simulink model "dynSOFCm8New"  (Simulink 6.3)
settings: Solver=ode15s  StartTime=0.0  StopTime=5000  FixedStep=0.001  MinStep=1e-12  RelTol=1e-3
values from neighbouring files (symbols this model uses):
  C = 300e-2    (= 3)    [dynSOFC_par.m]
  Cpc = 740    [dynSOFC_par.m]
  Cpt = 1217.7    [dynSOFC_par.m]
  D_a = 0.273*2*r3    (= 0.006006)    [dynSOFC_par.m]
  D_c = 2*(r2-r1)    (= 0.00532)    [dynSOFC_par.m]
  delta = 5.67e-8    (= 5.67e-08)    [dynSOFC_par.m]
  Ea = 1.1e5    (= 110000)    [dynSOFC_par.m]
  Ec = 1.2e5    (= 120000)    [dynSOFC_par.m]
  Ems1 = 0.4    [dynSOFC_par.m]
  Ems2 = 0.9    [dynSOFC_par.m]
  F = 96487    [dynSOFC_par.m]
  F21 = 0.69    [dynSOFC_par.m]
  K = 10    [dynSOFC_par.m]
  L = 1.5    [dynSOFC_par.m]
  La = 0.1e-3    (= 0.0001)    [dynSOFC_par.m]
  Lc = 2.21e-3    (= 0.00221)    [dynSOFC_par.m]
  Le = 0.04e-3    (= 4e-05)    [dynSOFC_par.m]
  R = 8.314/101325    (= 8.20528003948e-05)    [dynSOFC_par.m]
  r0 = 5e-3    (= 0.005)    [dynSOFC_par.m]
  r1 = 6e-3    (= 0.006)    [dynSOFC_par.m]
  r2 = 8.66e-3    (= 0.00866)    [dynSOFC_par.m]
  r3 = 11e-3    (= 0.011)    [dynSOFC_par.m]
  Ro = 1e-6    (= 1e-06)    [dynSOFC_par.m]
  Rouc = 4592    [dynSOFC_par.m]
  Rout = 3900    [dynSOFC_par.m]
  X = z(i)    [Simulate.m]    (also in dynSOFC_par.m = 0)
  x_ini = x_INI(i,:)    [Simulate.m]    (also in dynSOFC_par.m = [)
  XCH4 = 0.173    [dynSOFC_par.m]
  XCO = 0.057    [dynSOFC_par.m]
  XCO2 = 0.228    [dynSOFC_par.m]
  XH2 = 0.258    [dynSOFC_par.m]
  XH2O = 0.284    [dynSOFC_par.m]
  XO2 = 0.21    [dynSOFC_par.m]
libraries: simulink x23
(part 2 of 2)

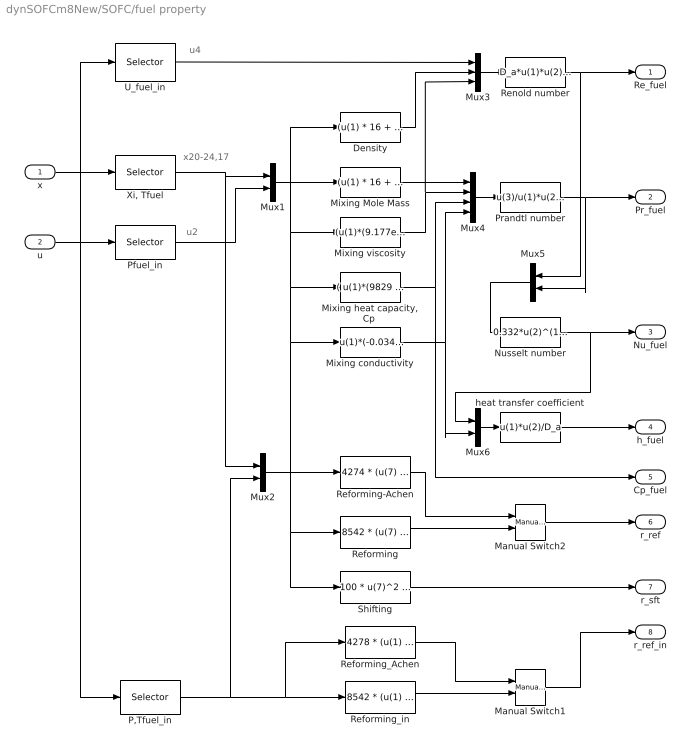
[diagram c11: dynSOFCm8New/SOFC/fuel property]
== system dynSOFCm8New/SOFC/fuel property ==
  note: x20-24,17
  note: u4
  note: u2
  x : Inport
  u : Inport  Port=2
  Density : Fcn  Expr="(u(1) * 16 + u(2) * 18 + u(3) * 2 + u(4) *28 + u(5) *44)  * u(7)/(R*u(6)) / 1000"
  Manual Switch1 : simulink/Signal Routing/Manual Switch  sw=0  action=0
  Manual Switch2 : simulink/Signal Routing/Manual Switch  sw=0  action=0
  Mixing Mole Mass : Fcn  Expr=(u(1) * 16 + u(2) * 18 + u(3) * 2 + u(4) *28 + u(5) *44)
  Mixing conductivity : Fcn  Expr=u(1)*(-0.03442 + 1.987e-4*u(6)) + u(2)*(-0.01450 + 9.782e-5*u(6)) + u(3)*(0.08525 + 2.964e-4*u(6)) + u(4)*(0.01275 + 5.348e-5*u(6)) + u(5)*(0.005485 + 6.272e-5*u(6))
  "Mixing heat capacity, Cp " : Fcn  Expr="( u(1)*(9829 + 83.47*u(6) -0.02053*u(6)^2)  + u(2)*(2.906e4 + 12.15*u(6)) +  u(3)*(2.660e4 +3.719*u(6)) + u(4)*(2.797e4 + 5.019*u(6)) + u(5)*(3.200e4 + 31.01*u(6) - 0.008875*u(6)^2) )"
  Mixing viscosity : Fcn  Expr="(u(1)*(9.177e-6 + 1.755e-8*u(6)) +  u(2)*(4.567e-6 + 2.209e-8*u(6)) + u(3)*(6.162e-6 + 1.145e-8*u(6)) + u(4)*(1.399e-5 + 2.582e-8*u(6)) + u(5)*(1.273e-5 + 2.822e-8*u(6)) )"
  Mux1 : Mux  Inputs=2
  Mux2 : Mux  Inputs=2
  Mux3 : Mux  Inputs=3
  Mux4 : Mux
  Mux5 : Mux  Orientation=left  Inputs=2
  Mux6 : Mux  Inputs=2
  Nusselt number : Fcn  Expr=0.332*u(2)^(1/3)*u(1)^(1/2)
  P,Tfuel_in : Selector  Elements=[2 3]  InputPortWidth=7
  Pfuel_in : Selector  Elements=[2]  InputPortWidth=7
  Prandtl number : Fcn  Expr=u(3)/u(1)*u(2)/u(4)
  Reforming : Fcn  Expr=8542 * (u(7) * u(1))^(0.85) * (u(7) * u(2))^(-0.35) * exp( -95e3 /(8.314*u(6)) )
  Reforming-Achen : Fcn  Expr=4274 * (u(7) * u(1)) * exp( -82e3 /(8.314*u(6)) )
  Reforming_Achen : Fcn  Expr=4278 * (u(1) * XCH4) * exp( -82e3 /(8.314*u(2)) )
  Reforming_in : Fcn  Expr=8542 * (u(1) * XCH4)^(0.85) * (u(1) * XH2O)^(-0.35) * exp( -95e3 /(8.314*u(2)) )
  Renold number : Fcn  Expr=D_a*u(1)*u(2)/u(3)
  Shifting : Fcn  Expr="100 * u(7)^2 * ( exp( 4276/u(6) - 3.961 ) * u(2) * u(4) -  u(3) * u(5) )"
  U_fuel_in : Selector  Elements=[4]  InputPortWidth=7
  "Xi, Tfuel" : Selector  Elements=[20 21 22 23 24 17]  InputPortWidth=25
  heat transfer coefficient : Fcn  Expr=u(1)*u(2)/D_a
  Re_fuel : Outport
  Pr_fuel : Outport  Port=2
  Nu_fuel : Outport  Port=3
  h_fuel : Outport  Port=4
  Cp_fuel : Outport  Port=5
  r_ref : Outport  Port=6
  r_sft : Outport  Port=7
  r_ref_in : Outport  Port=8
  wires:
  heat transfer coefficient/1 -> h_fuel/1
  Mux6/1 -> heat transfer coefficient/1
  Nusselt number/1 -> Mux6/1, Nu_fuel/1
  Mux5/1 -> Nusselt number/1
  Prandtl number/1 -> Mux5/2, Pr_fuel/1
  Mixing conductivity/1 -> Mux6/2, Mux4/4
  "Mixing heat capacity, Cp "/1 -> Mux4/3, Cp_fuel/1
  Mux4/1 -> Prandtl number/1
  Mixing viscosity/1 -> Mux4/2, Mux3/3
  Mixing Mole Mass/1 -> Mux4/1
  Renold number/1 -> Mux5/1, Re_fuel/1
  Mux3/1 -> Renold number/1
  Density/1 -> Mux3/2
  U_fuel_in/1 -> Mux3/1
  x/1 -> "Xi, Tfuel"/1
  "Xi, Tfuel"/1 -> Mux1/1, Mux2/1
  Mux1/1 -> Mixing Mole Mass/1, Mixing viscosity/1, "Mixing heat capacity, Cp "/1, Mixing conductivity/1, Reforming/1, Shifting/1, Density/1
  u/1 -> Pfuel_in/1, U_fuel_in/1, P,Tfuel_in/1
  Pfuel_in/1 -> Mux1/2
  P,Tfuel_in/1 -> Reforming_in/1, Reforming_Achen/1, Mux2/2
  Shifting/1 -> r_sft/1
  Manual Switch2/1 -> r_ref/1
  Reforming/1 -> Manual Switch2/2
  Reforming-Achen/1 -> Manual Switch2/1
  Manual Switch1/1 -> r_ref_in/1
  Reforming_Achen/1 -> Manual Switch1/1
  Reforming_in/1 -> Manual Switch1/2
  Mux2/1 -> Reforming-Achen/1

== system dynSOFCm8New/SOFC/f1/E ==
  x : Inport
  u : Inport  Port=2
  Constant : Constant  Orientation=up  Value=0
  E(t) : Display
  E0 : Fcn  Expr=1.2723-2.7645e-4*u(15)
  Eta_act2 : Display
  Eta_act_a+c : Fcn  Expr="2*8.314*u(4)/F/2 * (  log(u(3)/u(1)/2 +  (1+(u(3)/u(1)/2) ^2)^0.5  ) + log(u(3)/u(2)/2 +  (1+(u(3)/u(2)/2) ^2)^0.5 )/2   )"
  Iao : Display
  Ico : Display
  Manual Switch : simulink/Signal Routing/Manual Switch  Orientation=up  sw=1  action=0
  Mux : Mux
  Nernst : Fcn  Expr=8.314*u(15)/2/F*log(u(8)*(u(10)^0.5)/u(12))
  Nernst1 : Display
  Sum : Sum  Inputs=++-
  Tcell : Selector  Elements=[15]  InputPortWidth=25
  i : Selector  Elements=[1]  InputPortWidth=7
  ia0 : Fcn  Expr=7e9 * u(8) * u(12) * exp(-Ea/8.314/u(15))
  ic0 : Fcn  Expr=7e9 * (u(10)^0.25) * exp(-Ec/8.314/u(15) )
  E : Outport
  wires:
  Tcell/1 -> Mux/4
  Sum/1 -> E/1
  Eta_act_a+c/1 -> Eta_act2/1, Manual Switch/1
  Nernst/1 -> Sum/2, Nernst1/1
  E0/1 -> Sum/1, E(t)/1
  i/1 -> Mux/3
  u/1 -> i/1
  Mux/1 -> Eta_act_a+c/1
  ia0/1 -> Iao/1, Mux/1
  ic0/1 -> Mux/2, Ico/1
  x/1 -> ic0/1, ia0/1, Nernst/1, E0/1, Tcell/1
  Constant/1 -> Manual Switch/2
  Manual Switch/1 -> Sum/3
